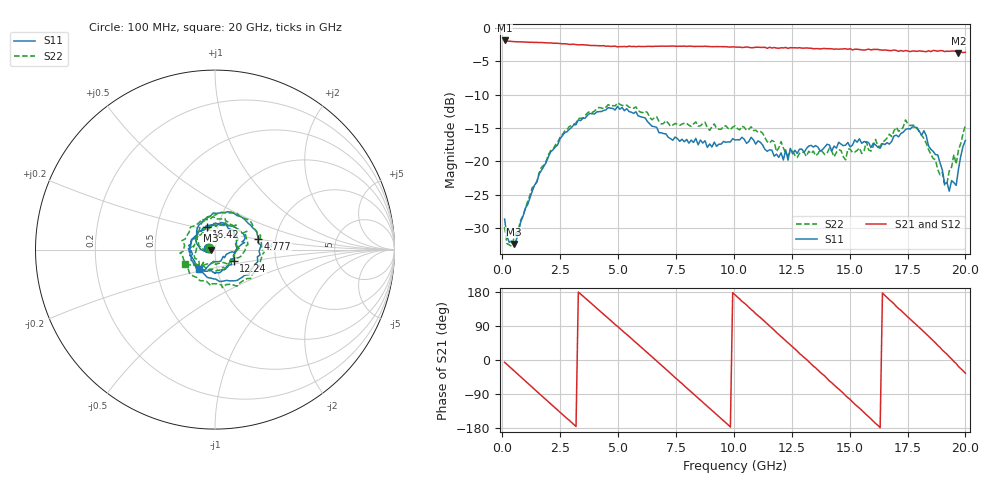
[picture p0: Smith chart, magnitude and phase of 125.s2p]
!Agilent Technologies,N5230C,MY49001569,A.09.33.09
!Agilent N5230C: A.09.33.09
!Date: Wednesday, July 29, 2015 19:31:46
!Correction: S11(Full 2 Port(1,2))
!S21(Full 2 Port(1,2))
!S12(Full 2 Port(1,2))
!S22(Full 2 Port(1,2))
!S2P File: Measurements: S11, S21, S12, S22:
# Hz S  dB  R 50
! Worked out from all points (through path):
!   201 points, 100 MHz to 20 GHz, reference 50 ohm
!   highest |S21| = -1.92 dB at 100 MHz (marker M1); lowest = -3.8 dB at 19.7 GHz (marker M2)
!   group delay of S21, straight-line fit = 154 ps
!   lowest |S11| = -32.3 dB at 498 MHz (marker M3), VSWR 1.05, Z = 47.7 - j0.457 ohm
!   |S11| at or under -10 dB: start of sweep to end of sweep
!   |S22| runs from -32.7 to -11.2 dB; largest |S21 - S12| = 0.023
!   S11 on the Smith chart (normalised r, x): 100 MHz: 0.93, +0.01; 4.777 GHz: 1.62, +0.21; 12.24 GHz: 1.22, -0.16; 16.42 GHz: 0.88, +0.23; 20 GHz: 0.81, -0.18
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1e8  -28.62 169.9  -1.92 -5.9  -1.89 -5.9  -29.81 168.7
4.98e8  -32.32 -168.6  -2.09 -28.2  -2.09 -28.1  -31.51 -172.3
1.7915e9  -20.76 167.9  -2.24 -99.3  -2.27 -99.3  -20.57 163.8
2.687e9  -15.73 123.6  -2.41 -148.3  -2.43 -148.3  -15.48 115.3
3.483e9  -13.57 79.5  -2.56 168.6  -2.57 168.6  -13.50 75.2
4.7765e9  -12.09 14.3  -2.79 99.3  -2.82 99.2  -11.66 8.6
5.672e9  -12.82 -30.3  -2.81 51.2  -2.84 51.4  -12.06 -35.9
6.7665e9  -15.70 -88.4  -2.78 -7.8  -2.75 -8.0  -14.02 -79.9
7.662e9  -16.99 -143.1  -2.77 -57.2  -2.79 -57.5  -14.63 -123.1
8.3585e9  -16.56 178.5  -2.81 -95.2  -2.84 -95.1  -14.10 -155.9
9.254e9  -17.75 126.1  -2.84 -144.1  -2.88 -144.4  -15.07 160.5
1.005e10  -16.80 83.4  -2.90 171.9  -2.92 172.2  -14.69 112.6
1.1244e10  -17.56 25.8  -2.96 106.5  -2.95 106.3  -15.78 49.0
1.2239e10  -18.27 -31.9  -2.97 50.9  -3.08 51.2  -18.77 -10.9
1.3433e10  -17.85 -91.3  -3.15 -16.0  -3.10 -15.1  -18.46 -86.8
1.4826e10  -17.56 -154.9  -3.16 -94.0  -3.25 -93.5  -19.77 174.4
1.6418e10  -17.32 109.5  -3.37 176.6  -3.38 175.9  -17.12 78.8
1.67165e10  -17.41 86.2  -3.43 159.0  -3.35 159.5  -15.92 69.3
1.81095e10  -16.10 16.3  -3.52 80.2  -3.56 78.7  -16.10 -8.0
1.91045e10  -23.36 -23.3  -3.58 20.9  -3.56 21.5  -23.54 -85.6
1.97015e10  -21.15 -109.2  -3.77 -17.1  -3.59 -15.5  -18.27 -130.5
2e10  -16.86 -129.8  -3.68 -34.9  -3.87 -35.2  -14.54 -153.8
